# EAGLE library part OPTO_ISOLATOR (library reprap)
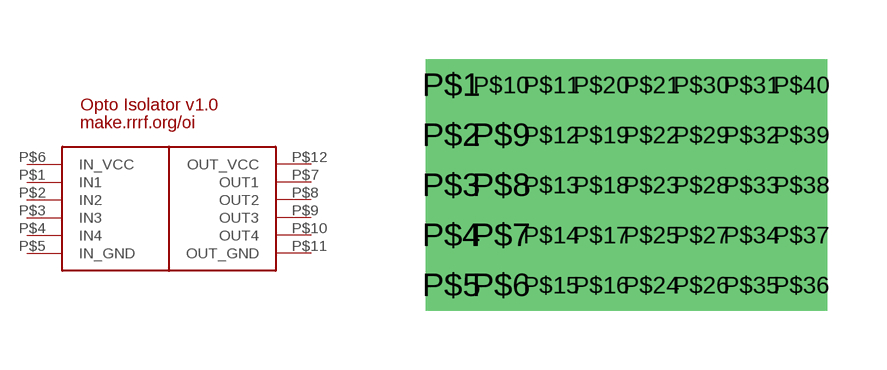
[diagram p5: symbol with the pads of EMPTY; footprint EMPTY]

Designator prefix -

## OPTO_ISOLATOR  [EMPTY]
P$1  IN1
P$2  IN2
P$3  IN3
P$4  IN4
P$5  IN_GND
P$6  IN_VCC
P$7  OUT1
P$8  OUT2
P$9  OUT3
P$10  OUT4
P$11  OUT_GND
P$12  OUT_VCC

## Footprint EMPTY (pad centres in mm)
drill 0.8 square: P$1 -1.27,5.08; P$2 -1.27,3.81; P$3 -1.27,2.54; P$4 -1.27,1.27; P$5 -1.27,0; P$6 0,0; P$7 0,1.27; P$8 0,2.54; P$9 0,3.81; P$10 0,5.08; P$11 1.27,5.08; P$12 1.27,3.81; P$13 1.27,2.54; P$14 1.27,1.27; P$15 1.27,0; P$16 2.54,0; P$17 2.54,1.27; P$18 2.54,2.54; P$19 2.54,3.81; P$20 2.54,5.08; P$21 3.81,5.08; P$22 3.81,3.81; P$23 3.81,2.54; P$24 3.81,0; P$25 3.81,1.27; P$26 5.08,0; P$27 5.08,1.27; P$28 5.08,2.54; P$29 5.08,3.81; P$30 5.08,5.08; P$31 6.35,5.08; P$32 6.35,3.81; P$33 6.35,2.54; P$34 6.35,1.27; P$35 6.35,0; P$36 7.62,0; P$37 7.62,1.27; P$38 7.62,2.54; P$39 7.62,3.81; P$40 7.62,5.08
